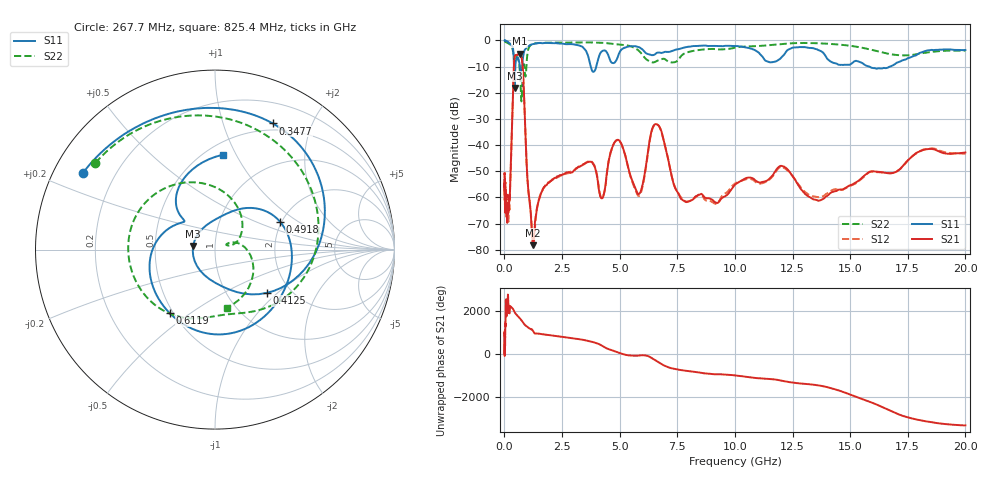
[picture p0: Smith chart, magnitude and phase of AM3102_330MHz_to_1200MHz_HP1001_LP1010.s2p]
! Date/Time: Tue, Sep 11, 2018 5:18 PM
! Network Analyzer: Agilent Technologies E8362B Rev: A.07.50.63
! Sweep from 0.010 to 20.000 GHz, 1601 Points, Sweep Type: LOG
! Power Supply: 4.949 V, 0.001 A
# Hz S DB R 50
!freq MagS11 AngS11 MagS21 AngS21 MagS12 AngS12 MagS22 AngS22
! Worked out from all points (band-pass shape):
!   1601 points, 10 MHz to 20 GHz, reference 50 ohm
!   highest |S21| = -5.01 dB at 663.4 MHz (marker M1); lowest = -78.3 dB at 1.224 GHz (marker M2)
!   |S21| within 3 dB of the highest: 424.2 MHz to 771.1 MHz (346.9 MHz wide, 58 % of centre)
!   lowest |S11| = -18.2 dB at 443 MHz (marker M3), VSWR 1.28, Z = 39.1 + j1.65 ohm
!   |S11| at or under -10 dB: 675.7 MHz to 769.5 MHz (93.75 MHz wide, 13 % of centre); 3.747 GHz to 3.985 GHz (237.8 MHz wide, 6.15 % of centre); 15.83 GHz to 16.73 GHz (894.8 MHz wide, 5.5 % of centre)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
!   |S22| runs from -23.3 to -0.2 dB; largest |S21 - S12| = 0.01
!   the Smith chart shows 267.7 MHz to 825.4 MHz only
!   S11 on the Smith chart (normalised r, x): 267.7 MHz: 0.09, +0.27; 347.7 MHz: 0.42, +1.47; 412.5 MHz: 1.52, -0.85; 491.8 MHz: 1.96, +0.72; 611.9 MHz: 0.48, -0.42; 825.4 MHz: 0.60, +0.89
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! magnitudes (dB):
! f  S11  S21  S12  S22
! 10 MHz  0.0  -51.1  -51.1  -0.2
! 35.55 MHz  0.0  -63.7  -63.7  -0.4
! 126.4 MHz  -0.4  -67.2  -63.5  -0.9
! 267.7 MHz  -1.4  -51.4  -52.1  -1.7
! 347.7 MHz  -2.2  -27.7  -27.8  -3.1
! 412.5 MHz  -8.5  -9.9  -9.9  -6.7
! 443 MHz  -18.2  -6.3  -6.4  -8.7
! 447.2 MHz  -18.0  -6.1  -6.2  -8.7
! 491.8 MHz  -8.1  -5.6  -5.6  -7.0
! 611.9 MHz  -7.2  -5.2  -5.3  -7.6
! 663.4 MHz  -9.2  -5.0  -5.1  -11.0
! 740 MHz  -12.4  -6.0  -6.1  -23.3
! 825.4 MHz  -5.5  -15.4  -15.5  -9.6
! 1.224 GHz  -1.4  -78.3  -76.9  -1.4
! 1.59 GHz  -1.0  -58.5  -58.2  -0.9
! 3.668 GHz  -7.2  -46.4  -46.1  -0.8
! 4.23 GHz  -4.2  -60.4  -60.2  -0.9
! 4.902 GHz  -6.8  -38.0  -38.1  -1.5
! 5.652 GHz  -2.2  -55.9  -56.6  -2.9
! 6.58 GHz  -4.9  -32.0  -32.1  -8.0
! 7.92 GHz  -2.5  -61.8  -61.7  -4.6
! 20 GHz  -3.6  -42.8  -43.3  -3.9
